{attribute 'no-analysis'}
FUNCTION_BLOCK FB_DirectControlEnhanced EXTENDS FB_DirectControl
VAR
END_VAR

METHOD Execute : BOOL
VAR
	bTestOk: BOOL; (*Used to cache the return value of the last '_OperativeTest' or '_DynamicTest' method call*)
	eError: E_AcsiServiceError; (*Used to cache the returned error of the last '_OperativeTest' or '_DynamicTest' method call*)
	tValue: T_UtcTime; (*Used to cache the current system time for 'tOpOk'*)
END_VAR
IF (_ipCtrl <> 0) AND_THEN (_ipCtrl.ipOper <> 0) THEN
	(* Initialize function block in the first cycle *)
	IF NOT bInit THEN
		_Init();
		bInit:=TRUE;
	END_IF

	CASE _eControlState OF
		E_DirectControlState.Ready:
			(* Check if ControlState changed in the last cycle *)
			IF bNewState THEN
				bNewState:=FALSE;
				_Reset();
			END_IF
			(* Check if a valid Oper_req was received *)
			IF bOperReq THEN
				bOperReq:=FALSE;
				(* Go to next ControlState *)
				_eControlState:=E_DirectControlState.PerformTest;
				bNewState:=TRUE;
			END_IF

		E_DirectControlState.PerformTest:
			(* Check if ControlState changed in the last cycle *)
			IF bNewState THEN
				bNewState:=FALSE;
				(* Set 'opRcvd' *)
				IF (_ipCtrl.ipOpRcvd <> 0) THEN
					_ipCtrl.ipOpRcvd.bValue:=TRUE;
				END_IF
			END_IF
			(* Trigger the operative test until it is finished *)
			IF _OperativeTest(bOperativeTestOk=>bTestOk, eError=>eError) THEN
				(* Reset 'opRcvd' *)
				IF (_ipCtrl.ipOpRcvd <> 0) THEN
					_ipCtrl.ipOpRcvd.bValue:=FALSE;
				END_IF
				IF bTestOk THEN
					(* Go to next ControlState *)
					_eControlState:=E_DirectControlState.WaitForExecution;
				ELSE
					fbCompletion.SetCompleted();
					fbCompletion.eServiceError:=eError;
					(* Go back to ControlState 'Ready' *)
					_eControlState:=E_DirectControlState.Ready;
				END_IF
				bNewState:=TRUE;
			END_IF

		E_DirectControlState.WaitForExecution:
			(* Check if ControlState changed in the last cycle *)
			IF bNewState THEN
				bNewState:=FALSE;
			END_IF
			(* Trigger the dynamic test until it is finished *)
			IF _DynamicTest(bDynamicTestOk=>bTestOk, eError=>eError) THEN
				fbCompletion.SetCompleted();
				IF bTestOk THEN
					(* Go to next ControlState *)
					IF (_ipBehVal <> 0) AND_THEN ((_ipBehVal.eValue = E_AcsiBeh.TestBlocked) OR_ELSE (_ipBehVal.eValue = E_AcsiBeh.OnBlocked)) THEN
						_eControlState:=E_DirectControlState.MirrorBlockedCommand;
					ELSE
						_eControlState:=E_DirectControlState.WaitForChange;
					END_IF
				ELSE
					fbCompletion.eServiceError:=eError;
					(* Go back to ControlState 'Ready' *)
					_eControlState:=E_DirectControlState.Ready;
				END_IF
				bNewState:=TRUE;
			END_IF

		E_DirectControlState.WaitForChange:
			(* Check if ControlState changed in the last cycle *)
			IF bNewState THEN
				bNewState:=FALSE;
				(* Set 'opOk' *)
				IF (_ipCtrl.ipOpOk <> 0) THEN
					_ipCtrl.ipOpOk.bValue:=TRUE;
				END_IF
				(* Set 'tOpOk' *)
				IF (_ipCtrl.ipTOpOk <> 0) AND_THEN (_ipCurrentAA <> 0) AND_THEN (_ipCurrentAA.GetSystemTime(tT=>tValue)) THEN
					_ipCtrl.ipTOpOk.tValue:=tValue;
				END_IF
			END_IF
			(* Update value *)
			_SetValue(uCtlVal:=_ipCtrl.ipOper.uCtlVal, ipCtlVal_AV:=_ipCtrl.ipOper.ipCtlVal_AnalogueValue);
			(* Update Timestamp 't' *)
			_UpdateTimestampValue(ipAA:=_ipCurrentAA);

			(* Reset 'opOk' *)
			IF (_ipCtrl.ipOpOk <> 0) THEN
				_ipCtrl.ipOpOk.bValue:=FALSE;
			END_IF
			(* Send CmdTerm_req+ *)
			_SendCommandTerminationReqPos(ipAA:=_ipCurrentAA, ipCtrlData:=_ipCtrl.ipOper);
			(* Go back to ControlState 'Ready' *)
			_eControlState:=E_DirectControlState.Ready;
			bNewState:=TRUE;

		E_DirectControlState.MirrorBlockedCommand:
			(* Check if ControlState changed in the last cycle *)
			IF bNewState THEN
				bNewState:=FALSE;
				(* Set 'opOk' *)
				IF (_ipCtrl.ipOpOk <> 0) THEN
					_ipCtrl.ipOpOk.bValue:=TRUE;
				END_IF
				(* Set 'tOpOk' *)
				IF (_ipCtrl.ipTOpOk <> 0) AND_THEN (_ipCurrentAA <> 0) AND_THEN (_ipCurrentAA.GetSystemTime(tT=>tValue)) THEN
					_ipCtrl.ipTOpOk.tValue:=tValue;
				END_IF
			END_IF
			(* Reset 'opOk' *)
			IF (_ipCtrl.ipOpOk <> 0) THEN
				_ipCtrl.ipOpOk.bValue:=FALSE;
			END_IF
			(* Send CmdTerm_req- *)
			_SendCommandTerminationReqNeg(ipAA:=_ipCurrentAA, ipCtrlData:=_ipCtrl.ipOper, eError:=E_AcsiApplError.NoError, ipOrigin:=_ipCtrl.ipOper.ipOrigin, ipCtlNum:=_ipCtrl.ipOper.ipCtlNum, eAddCause:=E_AcsiApplAddCause.BlockedByMode);
			(* Go back to ControlState 'Ready' *)
			_eControlState:=E_DirectControlState.Ready;
			bNewState:=TRUE;
	END_CASE
END_IF

(* Monitor transmission of LastApplError *)
CASE _nLastApplErrorReqState OF
	0:	;
	1:
		IF (_ipLastApplErrorReq <> 0) THEN
			Execute:=_ipLastApplErrorReq.Execute();
			IF NOT _ipLastApplErrorReq.IsBusy() THEN
				IF _ipLastApplErrorReq.IsCompleted() THEN
					SUPER^.SetCompleted();
				ELSE
					SUPER^.CopyFrom(ipSource:=_ipLastApplErrorReq);
				END_IF
				_nLastApplErrorReqState:=0;
			END_IF
		END_IF
END_CASE
(* Monitor transmission of CommandTermination *)
CASE _nCmdTermReqState OF
	0:	RETURN;
	1:
		IF (_ipCmdTermReq <> 0) THEN
			Execute:=_ipCmdTermReq.Execute();
			IF NOT _ipCmdTermReq.IsBusy() THEN
				IF _ipCmdTermReq.IsCompleted() THEN
					SUPER^.SetCompleted();
				ELSE
					SUPER^.CopyFrom(ipSource:=_ipLastApplErrorReq);
				END_IF
				_nCmdTermReqState:=0;
			END_IF
		END_IF
END_CASE
END_METHOD

END_FUNCTION_BLOCK
